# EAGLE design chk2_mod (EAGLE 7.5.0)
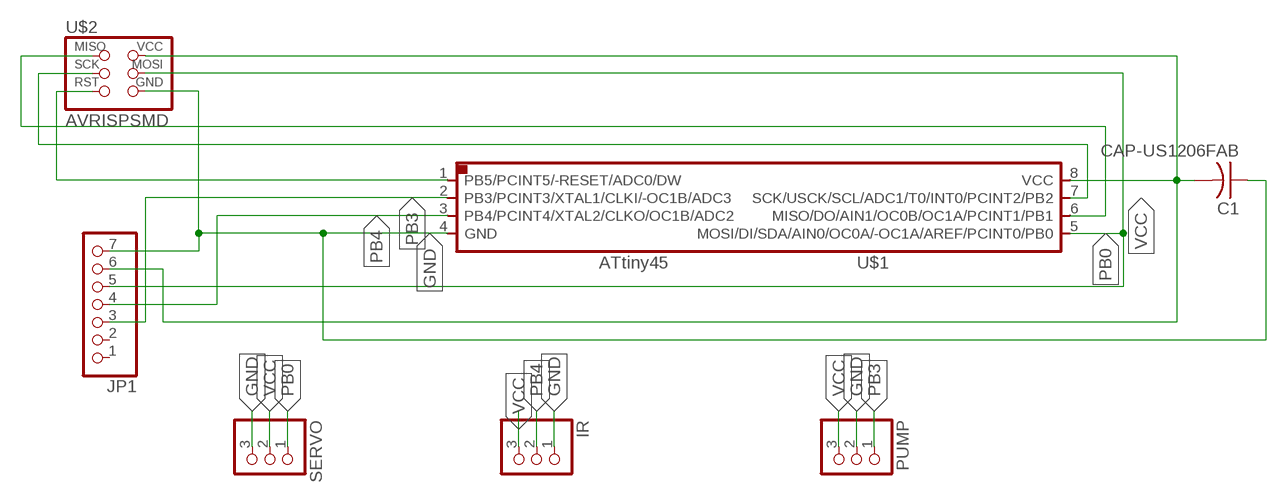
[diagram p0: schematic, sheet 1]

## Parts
C1  CAP-US1206FAB  [C1206FAB]
IR  PINHD-1X3  [1X03]
JP1  PINHD-1X7  [1X07]
PUMP  PINHD-1X3  [1X03]
SERVO  PINHD-1X3  [1X03]
U$1  ATTINY45SI  [SOIC8]
U$2  AVRISPSMD  [2X03SMD]

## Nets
GND: C1.1 IR.1 JP1.7 PUMP.2 SERVO.3 U$1.4(GND) U$2.6(GND)
N$3: U$1.6(MISO/DO/AIN1/OC0B/OC1A/PCINT1/PB1) U$2.1(MISO)
N$4: U$1.7(SCK/USCK/SCL/ADC1/T0/INT0/PCINT2/PB2) U$2.3(SCK)
N$6: U$1.1(PB5/PCINT5/-RESET/ADC0/DW) U$2.5(RST)
PB0: JP1.5 SERVO.1 U$1.5(MOSI/DI/SDA/AIN0/OC0A/-OC1A/AREF/PCINT0/PB0) U$2.4(MOSI)
PB3: JP1.3 PUMP.1 U$1.2(PB3/PCINT3/XTAL1/CLKI/-OC1B/ADC3)
PB4: IR.2 JP1.4 U$1.3(PB4/PCINT4/XTAL2/CLKO/OC1B/ADC2)
VCC: C1.2 IR.3 JP1.6 PUMP.3 SERVO.2 U$1.8(VCC) U$2.2(VCC)
Unconnected: JP1.1 JP1.2

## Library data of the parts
C1 = fab:CAP-US
IR PUMP SERVO = pinhead:PINHD-1X3: PIN HEADER
JP1 = pinhead:PINHD-1X7: PIN HEADER
U$1 = fab:ATTINY45
U$2 = fab:AVRISP

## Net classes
0 default: width 0.406 mm, drill 0.406 mm, clearance 0.406 mm

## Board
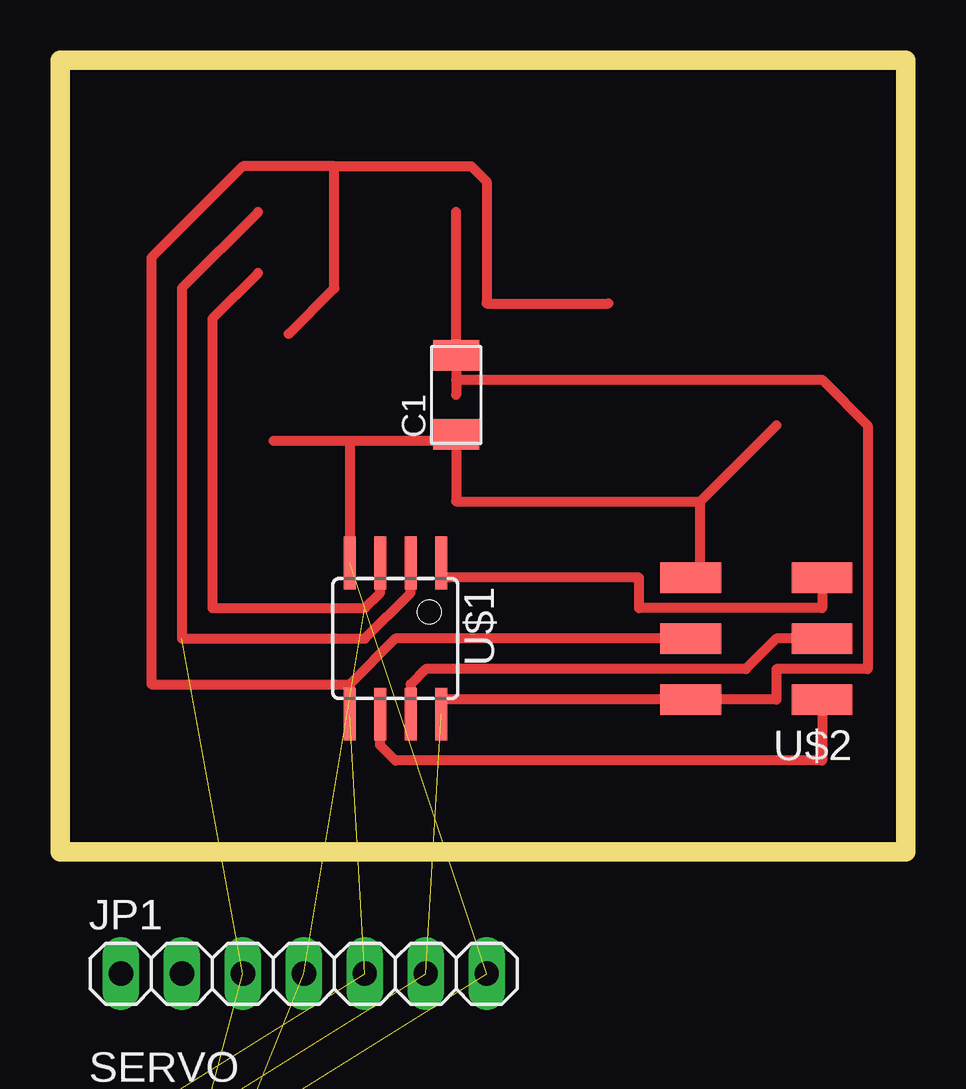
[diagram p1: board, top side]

Size 35.23 x 33.01 mm. Coordinates in mm from the lower left corner, seen from the top.
Outline: 0,0 35.23,0 35.23,33.01 0,33.01 0,0
Copper layers (1*16): Top 0.035mm / dielectric 1.5mm / Bottom 0.035mm
Design rules "default *": minimum track width 10mil, minimum drill 24mil, track to track 17mil, track to pad 17mil, pad to pad 17mil, via to via 17mil, smd to smd 8mil, copper to edge 40mil, drill to drill 8mil, minimum pad ring 10mil, minimum via ring 8mil, stop-mask expansion 4mil, vias tented up to drill 0mil, thermal gap 10mil

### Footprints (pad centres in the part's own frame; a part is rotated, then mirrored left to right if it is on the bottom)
C1206FAB = smd 1.27 x 1.905: 1 -1.651,0; 2 1.651,0
1X03 = drill 1.016 long: 1 -2.54,0; 2 0,0; 3 2.54,0
1X07 = drill 1.016 long: 1 -7.62,0; 2 -5.08,0; 3 -2.54,0; 4 0,0; 5 2.54,0; 6 5.08,0; 7 7.62,0
SOIC8 = smd 0.5 x 2.2: 1 -1.905,-3.154; 2 -0.645,-3.154; 3 0.625,-3.154; 4 1.895,-3.154; 5 1.905,3.154; 6 0.635,3.154; 7 -0.635,3.154; 8 -1.905,3.154
2X03SMD = smd 2.54 x 1.27: 1 -2.54,2.54; 2 2.92,2.54; 3 -2.54,0; 4 2.92,0; 5 -2.54,-2.54; 6 2.92,-2.54

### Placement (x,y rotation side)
C1  16.51,19.05 90 top
IR  not placed on the board
JP1  not placed on the board
PUMP  not placed on the board
SERVO  not placed on the board
U$1  13.97,8.89 180 top
U$2  29.21,8.89 180 top

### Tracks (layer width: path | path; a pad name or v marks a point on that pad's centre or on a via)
GND  (4 unrouted)
  Top 0.406: 26.67,14.61 29.85,17.78 | 26.67,14.61 26.67,11.43 U$2.6 | 8.89,17.15 12.06,17.15 | 12.06,17.15 16.51,17.15 | 12.06,17.15 12.06,12.07 U$1.4 | 26.67,14.61 16.51,14.61 16.51,17.15 | 16.51,17.15 C1.1
N$3
  Top 0.406: U$1.6 13.33,4.45 13.97,3.81 31.75,3.81 U$2.1
N$4
  Top 0.406: U$1.7 14.61,6.98 15.24,7.62 28.57,7.62 29.85,8.89 U$2.3
N$6
  Top 0.406: U$2.5 31.75,10.16 24.13,10.16 24.13,11.43 15.88,11.43 U$1.1
PB0  (2 unrouted)
  Top 0.406: 12.06,6.98 U$1.5 | 12.06,6.98 13.97,8.89 U$2.4 | 22.86,22.86 17.78,22.86 17.78,27.94 17.14,28.58 11.43,28.58 | 11.43,28.58 11.43,23.5 9.52,21.59 | 12.06,6.98 3.81,6.98 3.81,24.77 7.62,28.58 11.43,28.58
PB3  (2 unrouted)
  Top 0.406: 8.25,26.67 5.08,23.5 5.08,8.89 12.7,8.89 14.61,10.8 14.61,11.43 U$1.2
PB4  (2 unrouted)
  Top 0.406: 8.25,24.13 6.35,22.23 6.35,10.16 12.7,10.16 13.33,10.8 13.33,11.43 U$1.3
VCC  (4 unrouted)
  Top 0.406: U$1.8 15.88,6.35 U$2.2 29.85,6.35 29.85,7.62 33.66,7.62 33.66,17.78 31.75,19.69 16.51,19.69 | 16.51,26.67 C1.2 16.51,19.69 | 16.51,19.69 16.51,19.05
